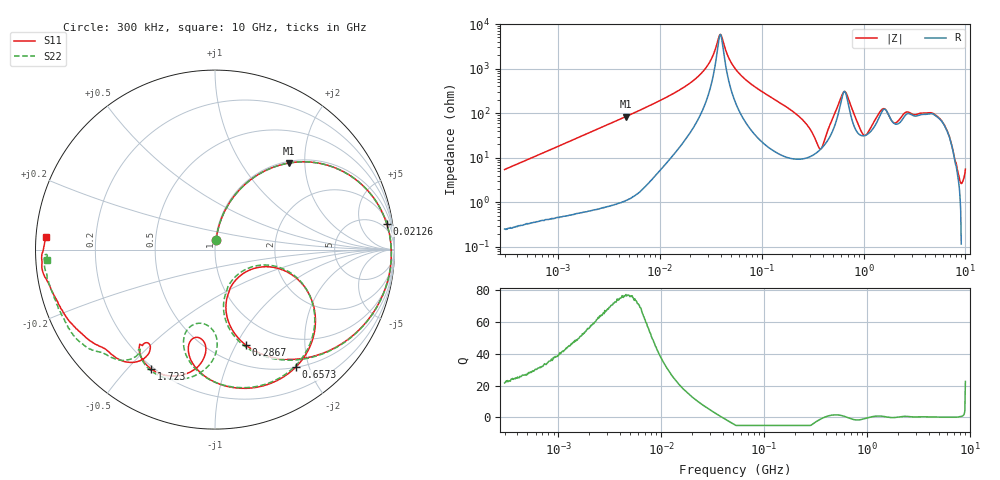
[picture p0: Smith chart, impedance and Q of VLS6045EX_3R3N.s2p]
! S-Parameter Data Generated by TDK Corporation
! Copyright(C) 2019 TDK Corporation.
! All Rights Reserved.
! TDK P/N: VLS6045EX-3R3N (Inductor)
! Property: L=3.3uH at 100kHz
! Size(LxWxT): 6x6x4.5mm
! Model Type: s2p (Touchstone File Format Version 1.0)
! Frequency: DC=Yes Start=0.3MHz Stop=10000MHz 802points Log-sweep
! Model Generated on May 10, 2019
! Port Assignments:
!  1 ---@@@--- 2
! Applicable Conditions:
!  Temperature = 25 degC
!  DC Bias Current = 0 A
!  Small Signal Operation
! Terms and conditions regarding TDK Simulation Models
! (1)This simulation model is being provided solely for informational purposes. Please refer to the specifications of the products in terms of detailed characteristics of such products.
! (2)In no event shall TDK Corporation of any of its subsidiaries be liable for any loss or damage arising, directly or indirectly,
!  From any information contained in this simulation model, including, but not limited to loss or damages arising from any inaccuracies, omissions or errors in connection with such information.
! (3)Any and all copyrights on this simulation model are owned by TDK Corporation.
!  Duplication or redistribution of this simulation model without prior written permission from TDK Corporation is prohibited.
! (4)This simulation model is subject to any modification or change without any prior notice.
! (5)Neither TDK Corporation nor any of its subsidiaries shall make any warranty, express or implied,
!  Including but not limited to the correctness, implied warranties of merchantability and fitness for a particular purpose with respect to this simulation models.
! (6)The use of this simulation model shall be deemed to have consented to the terms and conditions hereof.
# Hz S MA R 50
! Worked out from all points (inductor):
!   801 points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, 300 kHz to 10 GHz, reference 50 ohm
!   read as one part in series: L = 2.89 uH near 318.3 kHz
!   highest Q = 76.3 at 4.611 MHz (marker M1), where L = 2.87 uH
!   self-resonance near 39.05 MHz
!   S11 on the Smith chart (normalised r, x): 300 kHz: 1.01, +0.11; 21.26 MHz: 3, +13; 286.7 MHz: 0.71, -1.10; 657.3 MHz: 0.50, -1.79; 1.723 GHz: 0.19, -0.58; 10 GHz: 0.03, +0.04
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300000  0.0531 84.2  0.9959 -3.2  0.9962 -3.2  0.05311 84.0
1713600  0.29 71.9  0.9514 -17.0  0.9516 -17.0  0.29 71.9
4611084  0.6334 49.6  0.7656 -39.7  0.7655 -39.7  0.6335 49.6
9671944  0.8683 27.5  0.4742 -61.1  0.4741 -61.1  0.8684 27.4
2.126252e7  0.9677 8.6  0.1815 -76.4  0.1815 -76.4  0.9677 8.5
3.031424e7  0.9807 1.6  0.07571 -75.8  0.07572 -75.8  0.9808 1.6
3.904515e7  0.9831 -3.2  0.01691 -10.7  0.0169 -10.8  0.9833 -3.3
5.477226e7  0.978 -10.1  0.0962 69.4  0.09621 69.4  0.9781 -10.2
1.630679e8  0.8357 -43.5  0.4964 42.5  0.4963 42.5  0.8358 -44.0
2.867479e8  0.5593 -72.1  0.7526 9.1  0.7526 9.1  0.5581 -73.3
3.126428e8  0.4887 -76.4  0.7852 2.0  0.7851 2.0  0.4867 -77.8
4.20949e8  0.2042 -54.6  0.8096 -30.3  0.8096 -30.3  0.1909 -56.4
4.807079e8  0.3248 -17.3  0.709 -50.0  0.709 -50.0  0.3144 -16.0
6.573376e8  0.7944 -55.5  0.2025 -41.3  0.2027 -41.3  0.7895 -56.1
7.956093e8  0.7733 -82.9  0.3919 -16.4  0.392 -16.4  0.7635 -84.8
1.069912e9  0.549 -105.4  0.5774 -53.6  0.5779 -53.6  0.4973 -109.6
1.371335e9  0.607 -95.9  0.3973 -96.8  0.3987 -96.8  0.5467 -88.9
1.723085e9  0.7542 -118.2  0.2241 -84.3  0.2251 -84.6  0.7682 -112.5
1.767019e9  0.7471 -120.8  0.2331 -83.0  0.2341 -83.3  0.7674 -115.4
2.172958e9  0.6405 -125.7  0.2679 -108.4  0.2685 -109.0  0.6941 -126.9
6.818311e9  0.946 -168.4  0.03433 -148.2  0.0338 -147.6  0.9404 -167.3
1e10  0.9456 175.9  0.03314 -139.2  0.03354 -138.8  0.9389 -176.5
